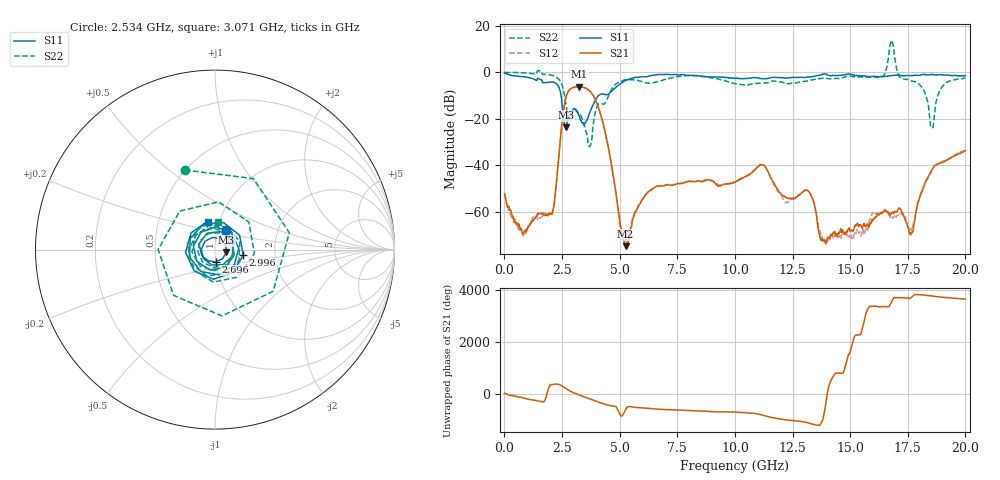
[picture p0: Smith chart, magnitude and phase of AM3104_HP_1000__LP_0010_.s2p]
!Created with skrf (http://scikit-rf.org).
# Hz S RI R 50.0
!freq ReS11 ImS11 ReS21 ImS21 ReS12 ImS12 ReS22 ImS22
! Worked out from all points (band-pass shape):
!   1601 points, 10 MHz to 20 GHz, reference 50 ohm
!   highest |S21| = -6.15 dB at 3.246 GHz (marker M1); lowest = -74.8 dB at 5.257 GHz (marker M2)
!   |S21| within 3 dB of the highest: 2.727 GHz to 3.8 GHz (1.074 GHz wide, 32.9 % of centre)
!   lowest |S11| = -23.7 dB at 2.671 GHz (marker M3), VSWR 1.14, Z = 56.7 - j1.83 ohm
!   |S11| at or under -10 dB: 2.46 GHz to 4.083 GHz (1.623 GHz wide, 49.6 % of centre)
!   |S22| runs from -31.9 to 13.7 dB; largest |S21 - S12| = 0.026
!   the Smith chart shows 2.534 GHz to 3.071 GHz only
!   S11 on the Smith chart (normalised r, x): 2.534 GHz: 1.10, +0.24; 2.696 GHz: 1.00, -0.14; 2.996 GHz: 1.37, -0.09; 3.071 GHz: 0.88, +0.28
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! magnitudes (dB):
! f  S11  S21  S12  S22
! 10 MHz  -0.3  -52.3  -52.1  0.0
! 834.6 MHz  -1.9  -69.0  -69.8  -0.2
! 2.046 GHz  -4.2  -61.0  -61.6  -1.2
! 2.534 GHz  -18.1  -18.8  -18.9  -6.5
! 2.671 GHz  -23.7  -10.8  -10.8  -14.0
! 2.696 GHz  -23.2  -10.0  -10.0  -15.7
! 2.996 GHz  -15.9  -6.5  -6.5  -16.7
! 3.071 GHz  -15.8  -6.3  -6.3  -16.3
! 3.246 GHz  -18.9  -6.2  -6.2  -17.9
! 3.346 GHz  -21.4  -6.3  -6.4  -19.2
! 3.708 GHz  -17.3  -8.0  -8.1  -31.9
! 4.195 GHz  -9.4  -18.8  -18.8  -13.5
! 5.257 GHz  -3.6  -74.8  -72.2  -3.1
! 6.682 GHz  -1.0  -48.9  -48.9  -4.0
! 10.01 GHz  -2.6  -47.4  -47.4  -4.9
! 13.34 GHz  -2.0  -53.8  -53.8  -3.3
! 13.85 GHz  -0.8  -72.4  -71.9  -2.5
! 16.68 GHz  -1.5  -60.6  -61.5  7.2
! 17.66 GHz  -1.5  -69.4  -67.4  -3.8
! 18.54 GHz  -0.9  -42.1  -42.1  -24.0
! 19 GHz  -1.2  -38.8  -38.4  -6.2
! 20 GHz  -1.4  -33.8  -33.7  -2.4
